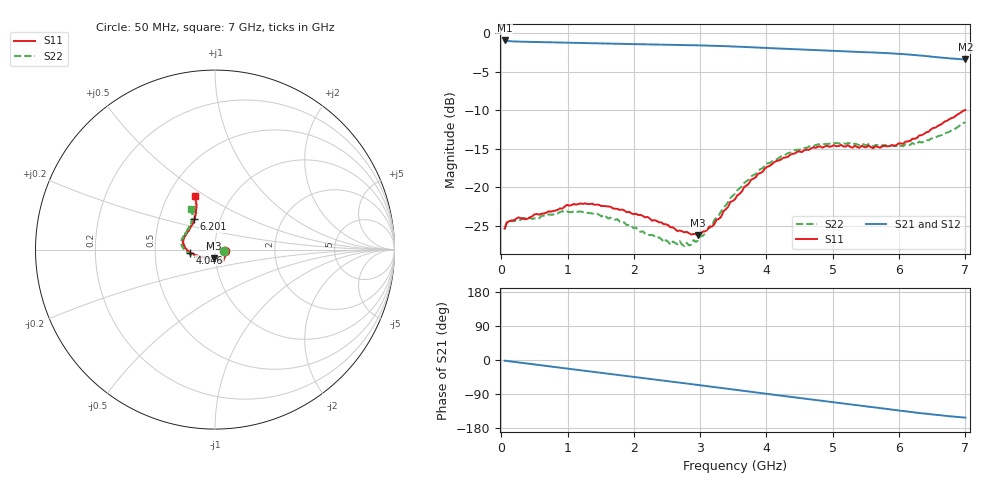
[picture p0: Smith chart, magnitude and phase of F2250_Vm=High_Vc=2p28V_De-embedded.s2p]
! Integrated Device Technology
! Corporate Headquarters
! 6024 Silver Creek Valley Road
! San Jose, CA 95138  USA
! Phone:  1-408-284-8200
! Toll Free:  1-800-223-1366
! Webpage:  http://www.idt.com/
! Timing and RF Division
! 515 Groton Road, Suite 102
! Westford, MA 01886-6024
! Device:  F2250
! Description: Voltage Variable RF Attenuator
! Frequency:  50.0 -  6000.00 MHz
! Package:  3x3 mm Thin QFN Plastic Package: 16 pin
! Ports:  2 RF, 3 DC
!  Pin  1  = GND
!  Pin  2  = NC
!  Pin  3  = RF1  = Port 1
!  Pin  4  = NC
!  Pin  5  = GND
!  Pin  6  = GND
!  Pin  7  = GND
!  Pin  8  = GND
!  Pin  9  = NC
!  Pin 10  = RF2  = Port 2
!  Pin 11  = NC
!  Pin 12  = GND
!  Pin 13  = GND
!  Pin 14  = VCNTRL
!  Pin 15  = VDD
!  Pin 16  = VMODE
! Vcntrl:  2.280 Volts
! Vmode:  +3.300 Volts
! Vdd:  +3.30  Volts
! Current:  1.315 mA
! Data:  The device was measured on a the F2250 evaluation board which has
!  individual transmission lines to the RF pins.  Data was collected
!  using a calibrated network analyzer.  The evaluation board was
!  de-embedded using a TRL calibration technique.
!  The reference plane is the edge of the package pin.
! Misc:  SN 10
!  Action Tracker AT0258
! Date Measured:  2014-11-26
! Date:  2015-10-15  MJV
! Note:
!  Integrated Device Technology supplies this data as a sample of measured
!  data at the package pin for this product.  Your particular data for this
!  product may vary.
!  Data was taken at 25 degrees C.
!  Integrated Device Technology reserves the right to change this data at anytime.
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# GHz S dB R 50
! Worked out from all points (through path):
!   201 points, 50 MHz to 7 GHz, reference 50 ohm
!   highest |S21| = -0.91 dB at 50 MHz (marker M1); lowest = -3.4 dB at 7 GHz (marker M2)
!   group delay of S21, straight-line fit = 61.1 ps
!   lowest |S11| = -26.2 dB at 2.969 GHz (marker M3), VSWR 1.10, Z = 49.3 - j4.79 ohm
!   |S11| at or under -10 dB: start of sweep to 6.984 GHz
!   |S22| runs from -27.7 to -11.5 dB; largest |S21 - S12| = 0.002
!   S11 on the Smith chart (normalised r, x): 50 MHz: 1.11, -0.02; 4.046 GHz: 0.76, -0.03; 6.201 GHz: 0.75, +0.27; 7 GHz: 0.68, +0.45
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0.05  -25.32 -10.3  -0.91 -1.8  -0.91 -1.8  -25.49 -10.6
0.1195  -24.43 -9.9  -1.01 -3.2  -1.01 -3.2  -24.38 -8.7
0.91875  -22.78 -49.1  -1.19 -21.0  -1.19 -21.1  -23.11 -50.4
1.2315  -22.16 -56.8  -1.26 -27.9  -1.26 -27.9  -23.22 -60.9
1.75275  -22.81 -63.8  -1.35 -39.1  -1.35 -39.1  -24.14 -67.5
2.37825  -24.55 -63.6  -1.44 -52.8  -1.44 -52.8  -26.50 -67.3
2.552  -25.20 -68.4  -1.47 -56.7  -1.47 -56.7  -27.45 -73.8
2.691  -25.62 -76.2  -1.49 -59.8  -1.49 -59.8  -27.00 -81.3
2.7605  -25.85 -78.3  -1.51 -61.3  -1.51 -61.3  -27.65 -85.8
2.969  -26.24 -95.9  -1.54 -66.0  -1.55 -66.0  -26.92 -104.9
3.21225  -24.80 -125.9  -1.60 -71.5  -1.60 -71.5  -24.26 -129.8
3.4555  -21.90 -146.9  -1.68 -77.0  -1.68 -77.0  -21.36 -145.1
3.525  -21.57 -151.3  -1.70 -78.5  -1.70 -78.6  -20.84 -148.3
3.76825  -19.01 -163.7  -1.79 -84.0  -1.79 -84.0  -18.60 -159.3
4.04625  -17.23 -173.2  -1.90 -90.2  -1.90 -90.2  -16.87 -169.7
4.4285  -15.59 176.6  -2.05 -98.6  -2.06 -98.6  -15.14 178.9
4.7065  -14.81 169.7  -2.15 -104.8  -2.15 -104.8  -14.64 173.1
5.054  -14.66 161.5  -2.28 -112.5  -2.27 -112.5  -14.24 166.1
5.85325  -14.64 135.6  -2.58 -130.0  -2.58 -130.1  -14.64 147.3
6.20075  -13.69 124.0  -2.79 -137.7  -2.79 -137.8  -14.23 138.3
6.54825  -12.25 115.9  -3.06 -144.7  -3.06 -144.8  -13.57 126.9
7  -9.96 111.0  -3.39 -152.1  -3.40 -152.2  -11.54 120.7
